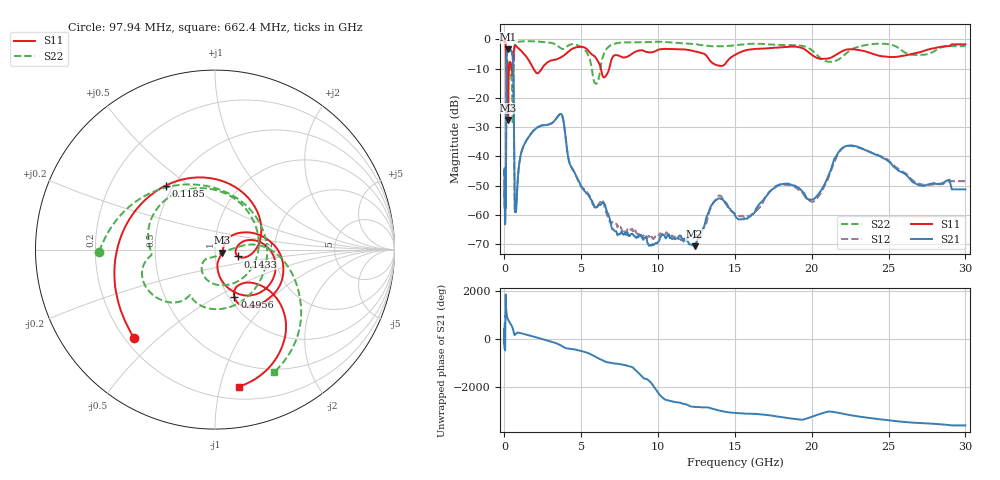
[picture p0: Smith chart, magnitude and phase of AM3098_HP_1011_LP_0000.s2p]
! Date/Time: Thu, Feb 28, 2019 8:42 AM
! Network Analyzer: Agilent Technologies E8364B Rev: A.07.50.67
! Sweep from 0.010 to 30.000 GHz, 1601 Points, Sweep Type: LOG
! Power Supply: 5.022 V, 0.002 A
# Hz S DB R 50
!freq MagS11 AngS11 MagS21 AngS21 MagS12 AngS12 MagS22 AngS22
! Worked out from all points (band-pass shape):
!   1601 points, 10 MHz to 30 GHz, reference 50 ohm
!   highest |S21| = -3.31 dB at 253.4 MHz (marker M1); lowest = -70.7 dB at 12.37 GHz (marker M2)
!   |S21| within 3 dB of the highest: 136.6 MHz to 538.8 MHz (402.2 MHz wide, 119 % of centre)
!   lowest |S11| = -27.5 dB at 239.9 MHz (marker M3), VSWR 1.09, Z = 54 - j1.75 ohm
!   |S11| at or under -10 dB: 200.2 MHz to 294.9 MHz (94.75 MHz wide, 38.3 % of centre); 1.888 GHz to 2.426 GHz (538 MHz wide, 24.9 % of centre); 6.274 GHz to 6.817 GHz (542.2 MHz wide, 8.28 % of centre)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
!   |S22| runs from -29.0 to -0.5 dB; largest |S21 - S12| = 0.01
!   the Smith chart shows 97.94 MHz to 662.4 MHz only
!   S11 on the Smith chart (normalised r, x): 97.94 MHz: 0.24, -0.42; 118.5 MHz: 0.46, +0.41; 143.3 MHz: 1.29, -0.10; 495.6 MHz: 1.06, -0.61; 662.4 MHz: 0.30, -1.14
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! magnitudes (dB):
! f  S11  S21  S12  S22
! 10 MHz  -0.3  -46.5  -44.4  -0.5
! 38.04 MHz  -0.4  -60.3  -59.8  -0.7
! 97.94 MHz  -3.5  -52.0  -52.5  -3.8
! 118.5 MHz  -6.9  -19.7  -19.7  -10.6
! 143.3 MHz  -17.4  -5.2  -5.2  -10.8
! 144.7 MHz  -18.1  -5.1  -5.0  -10.8
! 193.4 MHz  -9.2  -3.9  -3.8  -7.3
! 239.9 MHz  -27.5  -3.3  -3.3  -9.0
! 253.4 MHz  -20.7  -3.3  -3.3  -8.9
! 315.9 MHz  -8.5  -3.5  -3.5  -8.1
! 495.6 MHz  -10.9  -4.6  -4.5  -17.2
! 550.5 MHz  -11.2  -7.2  -7.2  -27.4
! 662.4 MHz  -2.2  -54.9  -55.9  -2.4
! 2.084 GHz  -11.5  -30.3  -30.3  -0.7
! 3.686 GHz  -6.1  -25.5  -25.5  -3.1
! 5.959 GHz  -6.4  -57.5  -57.5  -15.1
! 7.926 GHz  -6.0  -66.8  -65.9  -1.0
! 12.37 GHz  -4.1  -70.7  -67.8  -1.6
! 13.88 GHz  -8.9  -54.5  -53.6  -2.3
! 20.2 GHz  -5.9  -54.3  -55.1  -4.6
! 22.56 GHz  -3.3  -36.2  -36.4  -3.5
! 30 GHz  -1.7  -51.3  -48.5  -2.3
